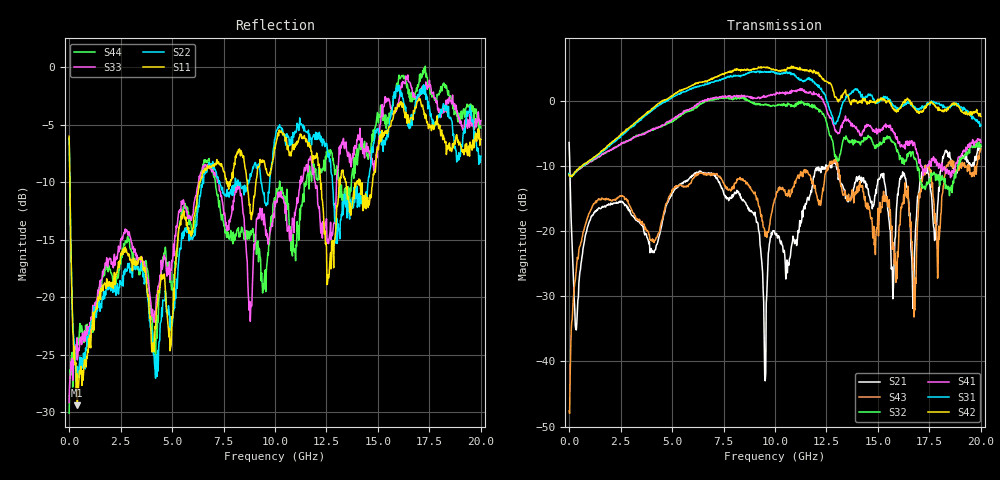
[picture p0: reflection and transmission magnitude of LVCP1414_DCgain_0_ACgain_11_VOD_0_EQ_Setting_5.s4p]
!Agilent Technologies,N5230A,MY46400459,A.07.50.48
!Agilent N5230A: A.07.50.48
!Date: Tuesday, April 17, 2012 18:42:57
!Correction: S11(Full 4 Port(1,2,3,4))
!S12(Full 4 Port(1,2,3,4))
!S13(Full 4 Port(1,2,3,4))
!S14(Full 4 Port(1,2,3,4))
!S21(Full 4 Port(1,2,3,4))
!S22(Full 4 Port(1,2,3,4))
!S23(Full 4 Port(1,2,3,4))
!S24(Full 4 Port(1,2,3,4))
!S31(Full 4 Port(1,2,3,4))
!S32(Full 4 Port(1,2,3,4))
!S33(Full 4 Port(1,2,3,4))
!S34(Full 4 Port(1,2,3,4))
!S41(Full 4 Port(1,2,3,4))
!S42(Full 4 Port(1,2,3,4))
!S43(Full 4 Port(1,2,3,4))
!S44(Full 4 Port(1,2,3,4))
!S4P File: Measurements: <S11,S12,S13,S14>,
!<S21,S22,S23,S24>,
!<S31,S32,S33,S34>,
!<S41,S42,S43,S44>:
# Hz S  dB  R 50
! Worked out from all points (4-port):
!   801 points, 300 kHz to 20 GHz, reference 50 ohm
!   strongest paths, dB at 300 kHz, 5 GHz, 10 GHz, 15 GHz, 20 GHz:
!     S42: -11.3, 0.8, 4.7, 0.2, -2.4
!     S31: -11.2, 0.5, 4.2, -0.2, -3.8
!     S41: -11.2, -2.8, 0.8, -4.5, -6.4
!     S32: -11.3, -3.3, -0.9, -7.0, -6.8
!     S43: -47.6, -13.7, -15.1, -16.5, -7.3
!     S21: -6.4, -14.1, -20.5, -12.1, -7.0
!   lowest |S11| = -29.4 dB at 400.3 MHz (marker M1), VSWR 1.07, Z = 53.1 + j1.52 ohm
!   |S11| at or under -10 dB: 37.56 MHz to 6.323 GHz (6.285 GHz wide, 198 % of centre); 12.21 GHz to 13.12 GHz (905.5 MHz wide, 7.15 % of centre); 14.13 GHz to 14.74 GHz (604.1 MHz wide, 4.19 % of centre)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
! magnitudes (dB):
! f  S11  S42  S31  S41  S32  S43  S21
! 300 kHz  -6.0  -11.3  -11.2  -11.2  -11.3  -47.6  -6.4
! 400.3 MHz  -29.4  -10.6  -10.6  -10.7  -10.7  -24.1  -32.3
! 6.25 GHz  -11.0  2.6  2.2  -0.6  -0.8  -11.4  -11.1
! 10.25 GHz  -5.6  4.6  4.0  1.1  -0.7  -13.6  -21.7
! 12.73 GHz  -17.5  2.5  -1.9  -2.8  -5.4  -9.7  -10.0
! 16.78 GHz  -3.9  -1.2  -0.9  -6.4  -9.0  -31.9  -23.6
! 20 GHz  -6.3  -2.4  -3.8  -6.4  -6.8  -7.3  -7.0
